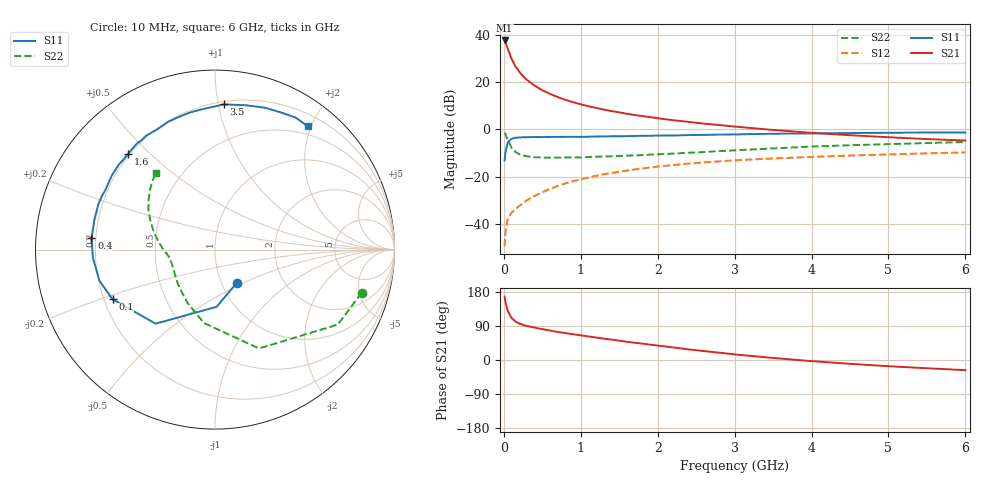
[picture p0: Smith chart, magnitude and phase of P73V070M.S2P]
! SIEMENS Small Signal Semiconductors
! BFP196
! Si NPN RF Bipolar Junction Transistor in SOT143
! VCE = 3 V  IC = 70 mA
! Common Emitter S-Parameters:  May  1996
# GHz  S  MA  R  50
!  f  S11  S21  S12  S22
! GHz  MAG  ANG  MAG  ANG  MAG  ANG  MAG  ANG
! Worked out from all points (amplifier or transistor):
!   36 points, 10 MHz to 6 GHz, reference 50 ohm
!   highest |S21| = 37.6 dB at 10 MHz (marker M1)
!   |S21| within 3 dB of that: start of sweep to 45.3 MHz
!   unconditionally stable (mu >= 1): 389 MHz to 4.436 GHz
!   at 250 MHz: K = 0.91, MSG = 26.8 dB, |S12| = -31.2 dB
!   at 1.4 GHz: K = 1.09, MAG = 11.3 dB, |S12| = -18.5 dB
!   at 6 GHz: K = 0.98, MSG = 2.5 dB, |S12| = -9.7 dB
!   S11 on the Smith chart (normalised r, x): 10 MHz: 1.18, -0.46; 100 MHz: 0.24, -0.22; 400 MHz: 0.18, +0.04; 1.6 GHz: 0.19, +0.43; 3.5 GHz: 0.22, +1.04; 6 GHz: 0.37, +1.95
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0.01  0.2215 -56.8  75.98 167.0  0.0034 79.0  0.8517 -16.4
0.02  0.3188 -88.4  70.09 154.4  0.0065 69.3  0.8016 -31.4
0.05  0.529 -128.7  51.21 129.8  0.0125 56.0  0.603 -66.0
0.1  0.6341 -154.1  31.1 110.8  0.0173 49.6  0.4136 -98.5
0.15  0.6668 -164.9  21.69 101.8  0.0205 52.6  0.3356 -116.7
0.2  0.6726 -171.7  16.58 96.3  0.024 55.9  0.2996 -128.6
0.25  0.682 -176.2  13.26 92.6  0.0276 58.4  0.2803 -137.6
0.3  0.6831 -179.7  11.13 89.8  0.0318 61.0  0.27 -143.3
0.4  0.6911 174.7  8.43 85.4  0.0393 63.2  0.2584 -151.8
0.5  0.6892 170.3  6.746 81.5  0.0468 64.6  0.2544 -157.5
0.6  0.6922 166.2  5.626 77.7  0.0553 65.2  0.2532 -161.1
0.7  0.6934 161.8  4.831 74.0  0.0637 65.0  0.2539 -164.0
0.9  0.6971 154.9  3.765 68.0  0.0804 63.5  0.2553 -168.3
1.1  0.7005 147.8  3.096 62.1  0.0961 61.3  0.2613 -171.4
1.3  0.7112 141.0  2.624 56.3  0.1126 58.7  0.2671 -174.1
1.6  0.7209 132.3  2.138 48.2  0.135 54.7  0.2792 -177.8
2.2  0.7429 115.8  1.565 33.2  0.1765 45.5  0.3078 174.5
2.8  0.776 100.6  1.237 19.3  0.2114 36.5  0.3479 165.5
3.5  0.8105 86.6  0.975 5.4  0.2435 26.4  0.397 155.4
4.5  0.838 70.6  0.754 -10.1  0.2799 14.4  0.4628 143.0
5.5  0.8619 58.6  0.625 -21.8  0.3116 3.6  0.5157 132.8
6  0.8598 53.0  0.582 -26.8  0.3264 -2.2  0.5404 127.7
